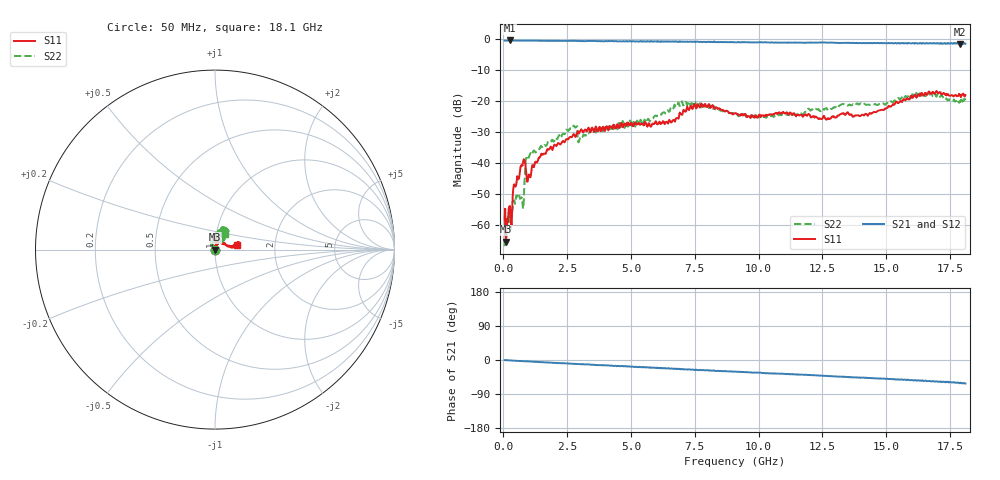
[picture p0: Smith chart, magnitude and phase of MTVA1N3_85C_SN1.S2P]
! Network Analyzer HP8720D.06.14 Serial No. US36140669
! 10 Jan 2005  15:16:48
! Frequency  S11  S21  S12  S22
# HZ  S  DB R 50
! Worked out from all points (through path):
!   801 points, 50 MHz to 18.1 GHz, reference 50 ohm
!   highest |S21| = -0.60 dB at 253.1 MHz (marker M1); lowest = -1.7 dB at 17.9 GHz (marker M2)
!   group delay of S21, straight-line fit = 9.1 ps
!   lowest |S11| = -65.3 dB at 95.12 MHz (marker M3), VSWR 1.00, Z = 50 + j0.0515 ohm
!   |S11| at or under -10 dB: start of sweep to end of sweep
!   |S22| runs from -66.8 to -17.4 dB; largest |S21 - S12| = 0.024
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5e7  -58.21 -77.3  -0.63 -0.3  -0.64 -0.4  -66.81 58.9
9.5125e7  -65.33 71.9  -0.66 -0.5  -0.65 -0.8  -62.14 -96.6
1.628125e8  -57.84 130.1  -0.64 -0.5  -0.65 -0.8  -58.47 157.7
2.530625e8  -53.87 119.8  -0.60 -1.0  -0.60 -1.2  -59.04 153.5
5.0125e8  -47.27 106.7  -0.64 -2.3  -0.64 -2.6  -50.69 120.5
7.494375e8  -40.88 84.4  -0.67 -2.9  -0.67 -3.2  -53.08 127.3
9.07375e8  -44.28 42.3  -0.65 -3.5  -0.65 -3.9  -37.75 167.1
9.750625e8  -44.68 73.9  -0.66 -3.8  -0.63 -4.0  -38.39 146.6
1.471438e9  -37.46 92.2  -0.70 -5.6  -0.68 -5.9  -34.54 124.0
2.689812e9  -31.67 74.6  -0.71 -9.8  -0.71 -10.2  -28.87 120.0
3.073375e9  -29.36 75.8  -0.78 -11.3  -0.75 -11.4  -31.81 128.2
6.074188e9  -27.42 80.0  -0.91 -21.6  -0.92 -21.6  -24.66 102.0
6.931562e9  -24.20 88.4  -0.98 -24.6  -0.98 -24.3  -21.33 83.8
7.54075e9  -22.37 80.2  -1.02 -25.3  -0.85 -26.3  -20.33 65.1
9.075e9  -23.99 91.0  -1.19 -30.7  -1.12 -31.1  -24.15 49.9
1.027081e10  -24.59 93.1  -1.16 -35.0  -1.20 -34.7  -25.41 51.3
1.209838e10  -25.19 70.2  -1.26 -39.9  -1.26 -40.2  -22.77 73.7
1.403875e10  -24.54 34.4  -1.48 -46.8  -1.44 -47.0  -20.95 74.9
1.509919e10  -21.64 14.4  -1.46 -50.4  -1.36 -50.1  -20.70 81.7
1.640781e10  -17.61 11.9  -1.60 -53.9  -1.46 -54.4  -18.27 65.9
1.789694e10  -18.04 11.2  -1.70 -60.0  -1.73 -60.6  -20.43 64.0
1.81e10  -18.18 12.8  -1.67 -62.1  -1.64 -63.2  -19.83 57.7
